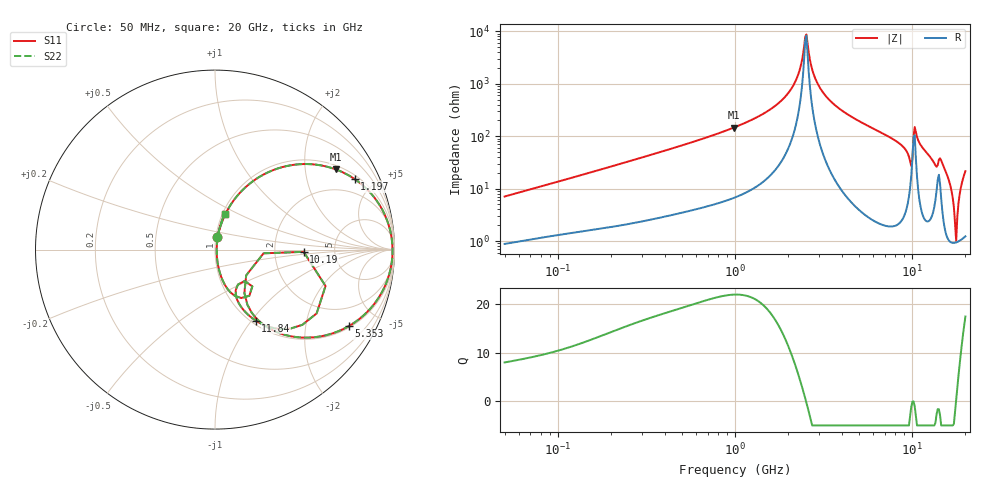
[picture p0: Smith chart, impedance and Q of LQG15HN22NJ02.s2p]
!Murata Part Number: LQG15HN22NJ02
!These Parameters are Measured in Series Mode Connection
!  o--[Z]--o
!Port1  Port2
!  o-------o
!Freq. Start=50[MHz] Stop=20[GHz], 401[Steps]
# Hz S RI R 50
!Freq.(Hz) S11(Real) S11(Imag) S21(Real) S21(Imag) S12(Real) S12(Imag) S22(Real) S22(Imag)
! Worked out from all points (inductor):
!   401 points, 50 MHz to 20 GHz, reference 50 ohm
!   read as one part in series: L = 22 nH near 51.52 MHz
!   highest Q = 21.9 at 985.1 MHz (marker M1), where L = 23.5 nH
!   self-resonance near 2.494 GHz
!   S11 on the Smith chart (normalised r, x): 50 MHz: 1.02, +0.14; 1.197 GHz: 1.18, +3.86; 5.353 GHz: 1.07, -3.45; 10.19 GHz: 2.95, -0.10; 11.84 GHz: 1.05, -1.05; 20 GHz: 1.02, +0.43
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5e7  0.0135 0.0685  0.9865 -0.0685  0.9865 -0.0685  0.0135 0.0685
1.364002e8  0.0455 0.1707  0.9545 -0.1707  0.9545 -0.1707  0.0455 0.1707
3.721004e8  0.2066 0.3776  0.7934 -0.3776  0.7934 -0.3776  0.2066 0.3776
9.85133e8  0.673 0.4469  0.327 -0.4469  0.327 -0.4469  0.673 0.4469
1e9  0.6814 0.4437  0.3186 -0.4437  0.3186 -0.4437  0.6814 0.4437
1.196911e9  0.778 0.3931  0.222 -0.3931  0.222 -0.3931  0.778 0.3931
2.021818e9  0.968 0.136  0.032 -0.136  0.032 -0.136  0.968 0.136
2.279204e9  0.9843 0.0627  0.0157 -0.0627  0.0157 -0.0627  0.9843 0.0627
2.493527e9  0.989 0.0061  0.011 -0.0061  0.011 -0.0061  0.989 0.0061
2.728004e9  0.987 -0.0511  0.013 0.0511  0.013 0.0511  0.987 -0.0511
3.415248e9  0.9514 -0.1927  0.0486 0.1927  0.0486 0.1927  0.9514 -0.1927
5.352748e9  0.7441 -0.427  0.2559 0.427  0.2559 0.427  0.7441 -0.427
7.442007e9  0.4818 -0.4899  0.5182 0.4899  0.5182 0.4899  0.4818 -0.4899
9.600142e9  0.1805 -0.307  0.8195 0.307  0.8195 0.307  0.1805 -0.307
1.019291e10  0.4939 -0.0124  0.5061 0.0124  0.5061 0.0124  0.4939 -0.0124
1.082228e10  0.4211 -0.4399  0.5789 0.4399  0.5789 0.4399  0.4211 -0.4399
1.183995e10  0.2268 -0.3955  0.7732 0.3955  0.7732 0.3955  0.2268 -0.3955
1.504638e10  0.0854 -0.2378  0.9146 0.2378  0.9146 0.2378  0.0854 -0.2378
1.646126e10  0.0216 -0.1086  0.9784 0.1086  0.9784 0.1086  0.0216 -0.1086
1.774144e10  0.00933 0.00334  0.9907 -0.00334  0.9907 -0.00334  0.00933 0.00334
1.912117e10  0.0265 0.124  0.9735 -0.124  0.9735 -0.124  0.0265 0.124
2e10  0.0544 0.2  0.9456 -0.2  0.9456 -0.2  0.0544 0.2
